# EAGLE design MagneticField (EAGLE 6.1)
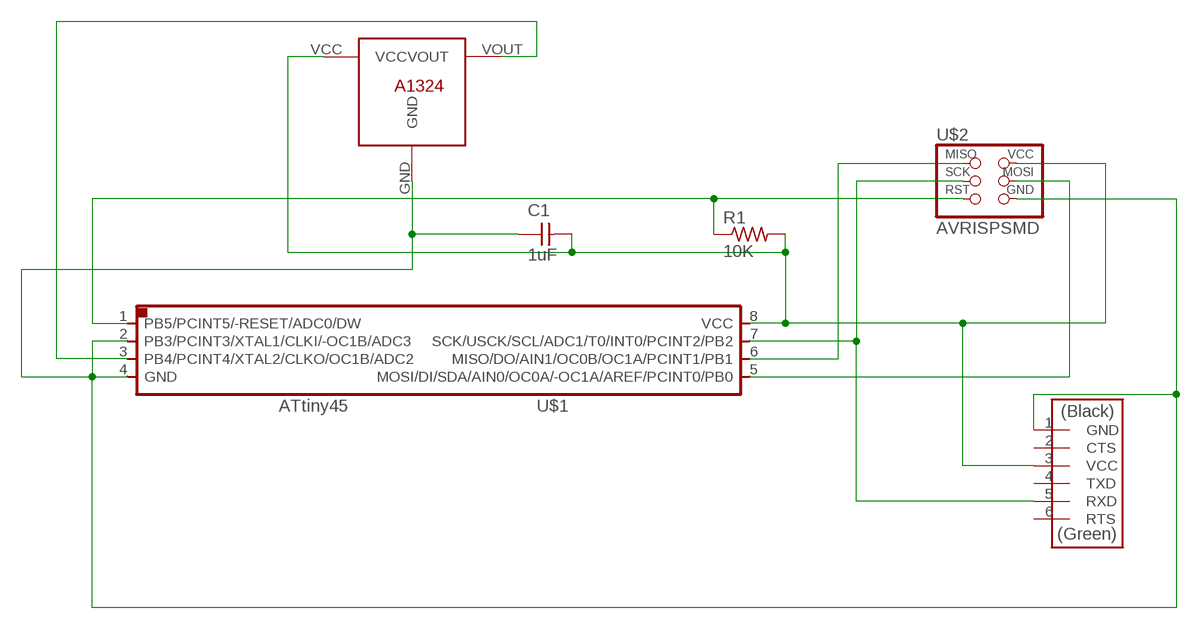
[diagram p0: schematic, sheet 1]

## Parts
C1  1uF  CAP-UNPOLARIZEDFAB  [C1206FAB]
R1  10K  RES-US1206FAB  [R1206FAB]
U$1  ATTINY45SI  [SOIC8]
U$2  AVRISPSMD  [2X03SMD]
U$3  FTDI-SMD-HEADER  [1X06SMD]
U$4  A1324_SMD  [A1324_SOT23W]

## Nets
GND: C1.1 U$1.2(PB3/PCINT3/XTAL1/CLKI/-OC1B/ADC3) U$1.4(GND) U$2.6(GND) U$3.1(GND) U$4.GND
N$1: U$1.7(SCK/USCK/SCL/ADC1/T0/INT0/PCINT2/PB2) U$2.3(SCK) U$3.5(RXD)
N$2: U$1.6(MISO/DO/AIN1/OC0B/OC1A/PCINT1/PB1) U$2.1(MISO)
N$3: U$1.5(MOSI/DI/SDA/AIN0/OC0A/-OC1A/AREF/PCINT0/PB0) U$2.4(MOSI)
N$4: R1.1 U$1.1(PB5/PCINT5/-RESET/ADC0/DW) U$2.5(RST)
N$9: U$1.3(PB4/PCINT4/XTAL2/CLKO/OC1B/ADC2) U$4.VOUT
VCC: C1.2 R1.2 U$1.8(VCC) U$2.2(VCC) U$3.3(VCC) U$4.VCC
Unconnected: U$3.2(CTS) U$3.4(TXD) U$3.6(RTS)

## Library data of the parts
C1 = fab:CAP-UNPOLARIZED
R1 = fab:RES-US: Resistor (US Symbol)
U$1 = fab:ATTINY45
U$2 = fab:AVRISP
U$3 = fab:FTDI-SMD-HEADER
U$4 = myFab:A1324_SMD

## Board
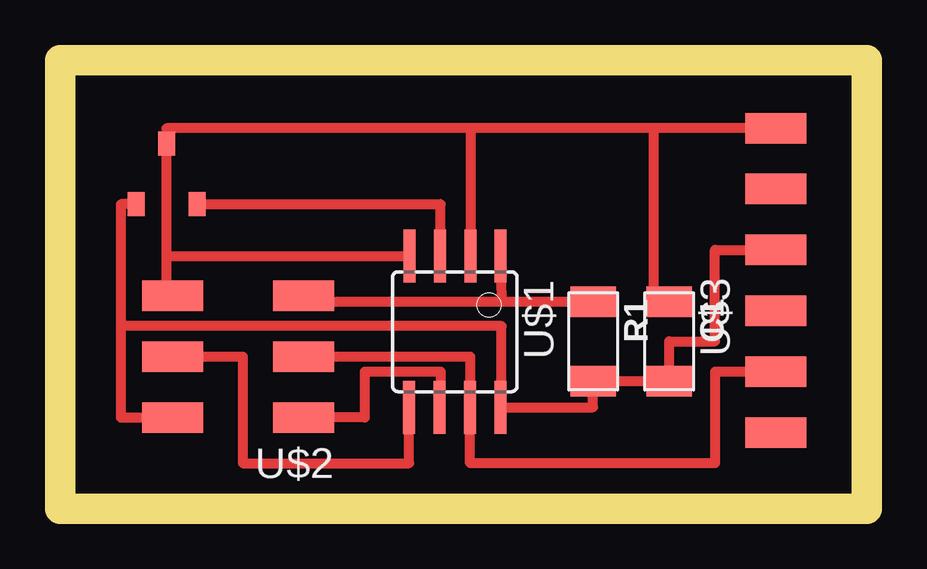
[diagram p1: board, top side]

Size 33.63 x 18.72 mm. Coordinates in mm from the lower left corner, seen from the top.
Outline: 0,0 33.63,0 33.63,18.72 0,18.72 0,0
Copper layers (1*16): Top 0.035mm / dielectric 1.5mm / Bottom 0.035mm
Design rules: minimum track width 10mil, minimum drill 24mil, track to track 8mil, track to pad 8mil, pad to pad 8mil, via to via 8mil, smd to smd 8mil, copper to edge 40mil, drill to drill 8mil, minimum pad ring 10mil, minimum via ring 8mil, stop-mask expansion 4mil, vias tented up to drill 0mil, thermal gap 10mil

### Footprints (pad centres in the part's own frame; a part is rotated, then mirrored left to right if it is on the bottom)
C1206FAB = smd 1.27 x 1.905: 1 -1.651,0; 2 1.651,0
R1206FAB = smd 1.27 x 1.905: 1 -1.651,0; 2 1.651,0
SOIC8 = smd 0.5 x 2.2: 1 -1.905,-3.154; 2 -0.645,-3.154; 3 0.625,-3.154; 4 1.895,-3.154; 5 1.905,3.154; 6 0.635,3.154; 7 -0.635,3.154; 8 -1.905,3.154
2X03SMD = smd 2.54 x 1.27: 1 -2.54,2.54; 2 2.92,2.54; 3 -2.54,0; 4 2.92,0; 5 -2.54,-2.54; 6 2.92,-2.54
1X06SMD = smd 2.54 x 1.27: 1 0,6.35; 2 0,3.81; 3 0,1.27; 4 0,-1.27; 5 0,-3.81; 6 0,-6.35
A1324_SOT23W = smd 0.7 x 1: GND 0,1.27; VCC -1.27,-1.27; VOUT 1.27,-1.27

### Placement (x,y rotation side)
C1  25.4,6.99 270 top
R1  22.23,6.99 270 top
U$1  16.46,7.38 180 top
U$2  7.62,6.35 180 top
U$3  29.84,9.53 0 top
U$4  4.45,13.97 0 top

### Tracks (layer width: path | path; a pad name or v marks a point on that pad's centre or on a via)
GND
  Top 0.406: U$3.1 24.77,15.88 | 24.77,15.88 17.14,15.88 | 17.14,15.88 4.45,15.88 U$4.GND 4.45,8.89 U$2.6 4.45,8.89 4.45,10.55 U$1.4 | C1.1 24.77,8.64 24.77,15.88 | U$1.2 17.14,10.54 17.14,15.88
N$1
  Top 0.406: U$2.3 17.09,6.35 U$1.7 17.09,1.91 27.3,1.91 27.3,5.71 U$3.5
N$2
  Top 0.406: U$1.6 15.88,4.23 15.88,5.71 12.7,5.71 12.7,3.81 U$2.1
N$3
  Top 0.406: U$2.4 7.62,6.35 7.62,1.91 14.55,1.91 U$1.5
N$4
  Top 0.406: U$2.5 11.15,8.89 11.15,8.64 | R1.1 18.41,8.64 | 18.41,8.64 11.15,8.64 | 11.15,8.64 11.15,8.55 | U$1.1 18.41,8.64
N$9
  Top 0.406: U$4.VOUT 15.84,12.7 | 15.88,12.7 15.84,12.7 | 15.84,12.7 U$1.3
VCC
  Top 0.406: U$4.VCC 2.54,12.7 2.54,7.62 | 2.54,7.62 2.54,3.81 U$2.2 | 2.54,7.62 18.41,7.62 18.41,4.23 U$1.8 22.23,4.23 R1.2 C1.2 25.4,6.99 27.3,6.99 27.3,10.79 U$3.3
